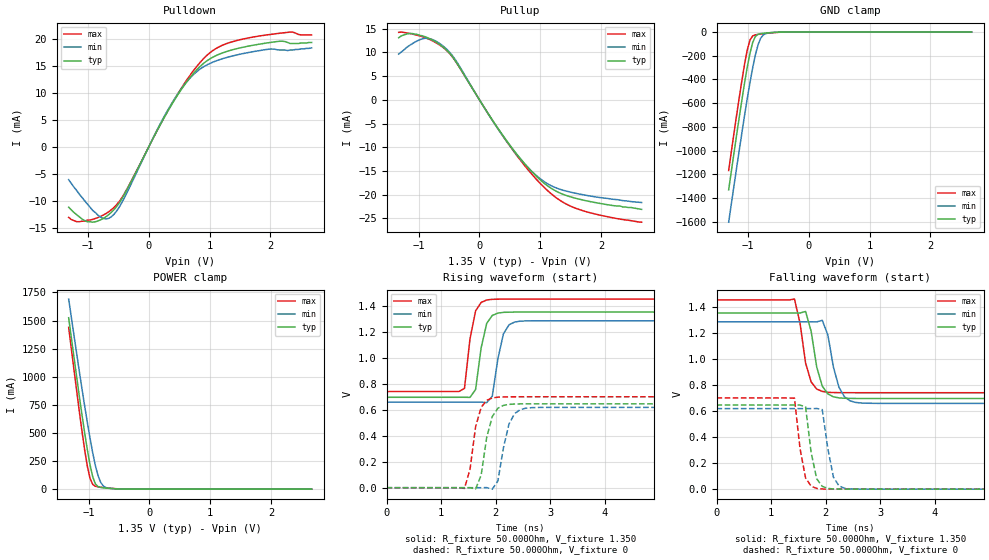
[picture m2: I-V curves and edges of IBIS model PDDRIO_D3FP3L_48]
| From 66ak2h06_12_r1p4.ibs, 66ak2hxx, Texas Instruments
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|   Model PDDRIO_D3FP3L_48
[Model] PDDRIO_D3FP3L_48
Model_type   I/O
Polarity   Non-Inverting
Enable   Active-High
C_comp   3.244pF   3.179pF   3.327pF
C_comp_pullup   525.014fF   499.307fF   553.259fF
C_comp_pulldown 2.714pF   2.675pF   2.768pF
Vinh = 810.000mV
Vinl = 540.000mV
Vmeas = 675.000mV
Vref = 675.000mV
Rref = 50Ohms
Cref = 0pF
[Model Spec]
Vinh   810.000mV   777.000mV   860.000mV
Vinl   540.000mV   507.000mV   590.000mV
Vmeas   675.000mV   642.000mV   725.000mV
Vref   675.000mV   642.000mV   725.000mV
[Temperature Range]   25.000   125.000   -40.000
[Voltage Range]   1.350V   1.283V   1.450V
[GND Clamp Reference]   0.00V   0.00V   0.00V
|[C Comp Corner]
| variable   typ   min   max
|C_comp 3.244pF   3.327pF   3.179pF
|C_comp_pullup 525.014fF   553.259fF   499.307fF
|C_comp_pulldown 2.714pF   2.768pF   2.675pF
[Pulldown Reference]   0.00V   0.00V   0.00V
[POWER Clamp Reference]   1.350V   1.283V   1.450V
[Pullup Reference]   1.350V   1.283V   1.450V
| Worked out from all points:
|   slope of the pulldown table from 0 to 0.203 V, typ, clamps not added: 46.1 ohm
|   slope of the pullup table from 0 to 0.203 V, typ, clamps not added: 49.9 ohm
|   GND clamp passes 1 mA (typ) near -0.49 V on its own axis
|   POWER clamp passes 1 mA (typ) near -0.46 V on its own axis
|   rising waveform, R_fixture 50.000Ohm, V_fixture 1.350: 20-80 % time 157ps typ, 163ps min, 148ps max; typ from 0.695 V to 1.35 V
|   rising waveform, R_fixture 50.000Ohm, V_fixture 0: 20-80 % time 172ps typ, 180ps min, 165ps max; typ from 0 V to 0.645 V
|   falling waveform, R_fixture 50.000Ohm, V_fixture 1.350: 20-80 % time 185ps typ, 193ps min, 181ps max; typ from 1.35 V to 0.695 V
|   falling waveform, R_fixture 50.000Ohm, V_fixture 0: 20-80 % time 145ps typ, 150ps min, 143ps max; typ from 0.645 V to 0 V
[GND Clamp]
-1.318V   -1.332A    -1.605A    -1.169A
-1.142V   -713.1mA   -991.3mA   -546.4mA
-1.055V   -424.6mA   -698mA     -266.3mA
-1.011V   -292.9mA   -557.9mA   -149mA
-966.7mV  -177mA     -424.6mA   -66.54mA
-922.7mV  -87.81mA   -301.3mA   -32.09mA
-878.8mV  -37.14mA   -193.2mA   -23.25mA
-834.9mV  -18.49mA   -107.6mA   -19.58mA
-790.9mV  -12.57mA   -51.47mA   -16.65mA
-747mV    -9.756mA   -23.13mA   -13.9mA
-439.4mV  -371uA     -394.7uA   -656.8uA
2.68V     4.17nA     252.6nA    785.5pA
[Power Clamp]
-1.33V    1.525A     1.691A     1.439A
-1.155V   827.2mA    1.048A     691.5mA
-1.067V   501.3mA    740.6mA    350.5mA
-1.023V   351.3mA    593.8mA    204.8mA
-978.8mV  217.4mA    454mA      97mA
-934.9mV  111.2mA    324.7mA    43.08mA
-890.9mV  47.28mA    211.3mA    25.9mA
-847mV    22.44mA    121mA      20.68mA
-803mV    14.88mA    60.26mA    17.58mA
-759.1mV  11.71mA    27.92mA    14.82mA
-407.6mV  326.5uA    576uA      395.5uA
2.668V    -7.545nA   -288.5nA   -3.819nA
[Pulldown]
-1.318V   -11.2mA    -6.1mA     -13.1mA
-1.011V   -13.9mA    -10.6mA    -13.6mA
-790.9mV  -13.54mA   -13.05mA   -12.9mA
-659.1mV  -12.59mA   -13.27mA   -12.05mA
-395.5mV  -8.712mA   -9.342mA   -8.569mA
351.5mV   7.366mA    7.581mA    7.447mA
790.9mV   14.34mA    13.99mA    14.96mA
1.098V    16.92mA    15.94mA    18.22mA
1.45V     18.25mA    17.09mA    19.77mA
2.153V    19.62mA    18mA       21.11mA
2.329V    19.2mA     18mA       21.33mA
2.68V     19.4mA     18.4mA     20.8mA
[Pullup]
-1.33V    13.1mA     9.662mA    14.24mA
-1.155V   14mA       11.46mA    14.03mA
-890.9mV  13.3mA     13mA       13.11mA
-583.3mV  10.99mA    11.18mA    10.9mA
-407.6mV  8.446mA    8.664mA    8.409mA
163.6mV   -3.298mA   -3.373mA   -3.333mA
515.1mV   -9.8mA     -9.916mA   -9.993mA
822.7mV   -14.62mA   -14.58mA   -15.1mA
1.13V     -18.22mA   -17.77mA   -19.25mA
1.394V    -20.01mA   -19.12mA   -21.74mA
1.658V    -20.99mA   -19.9mA    -23.2mA
2.668V    -23.1mA    -21.65mA   -25.8mA
[Ramp]
R_load=50.000Ohm
dV/dt_r   389.910mV/155.000ps  372.899mV/166.000ps  422.940mV/142.500ps
dV/dt_f   389.910mV/149.000ps  372.899mV/160.500ps  422.940mV/139.000ps
[Rising waveform]
R_fixture=50.000Ohm
V_fixture=1.350
V_fixture_min=1.283
V_fixture_max=1.450
0s        695mV      657.5mV    739.2mV
1.429ns   695.1mV    657.5mV    763.2mV
1.531ns   694.3mV    657.6mV    1.145V
1.633ns   754.4mV    657.6mV    1.359V
1.735ns   1.075V     657.5mV    1.424V
1.837ns   1.263V     653.9mV    1.443V
1.939ns   1.324V     703.1mV    1.448V
2.144ns   1.348V     1.183V     1.45V
2.348ns   1.35V      1.273V     1.45V
10ns      1.35V      1.283V     1.45V
[Rising waveform]
R_fixture=50.000Ohm
V_fixture=0
0s        0V         2.106uV    0V
1.429ns   657.3nV    -1.974uV   -5.646mV
1.531ns   194.2uV    4.452uV    141mV
1.633ns   -9.885mV   -741nV     467.8mV
1.735ns   95.78mV    8.031uV    617.2mV
1.939ns   547.2mV    -11.26mV   689.7mV
2.042ns   610.7mV    51.38mV    695.8mV
2.246ns   640.4mV    490mV      698.6mV
2.552ns   644.5mV    611.1mV    699mV
10ns      644.7mV    617.5mV    699mV
[Falling waveform]
R_fixture=50.000Ohm
V_fixture=1.350
V_fixture_min=1.283
V_fixture_max=1.450
0s        1.35V      1.283V     1.45V
1.429ns   1.35V      1.283V     1.457V
1.531ns   1.35V      1.283V     1.273V
1.633ns   1.362V     1.283V     966.8mV
1.735ns   1.21V      1.283V     821.8mV
1.837ns   936.5mV    1.282V     767.2mV
1.939ns   789.5mV    1.294V     749mV
2.246ns   699.6mV    779.8mV    739.6mV
2.552ns   695.3mV    664.9mV    739.2mV
10ns      695mV      657.5mV    739.2mV
[Falling waveform]
R_fixture=50.000Ohm
V_fixture=0
0s        644.7mV    617.5mV    699mV
1.429ns   644.7mV    617.5mV    697.5mV
1.531ns   644.7mV    617.5mV    310.8mV
1.633ns   630.7mV    617.5mV    85.38mV
1.735ns   280.3mV    617.5mV    22.86mV
1.837ns   79.32mV    618.2mV    5.881mV
1.939ns   21.61mV    609.8mV    1.538mV
2.144ns   1.462mV    91.38mV    92.16uV
2.348ns   97.43uV    6.922mV    3.016uV
10ns      0V         2.109uV    0V
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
